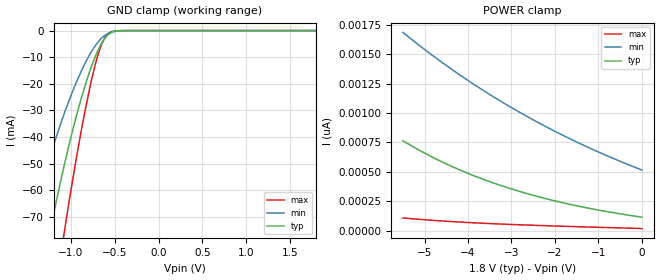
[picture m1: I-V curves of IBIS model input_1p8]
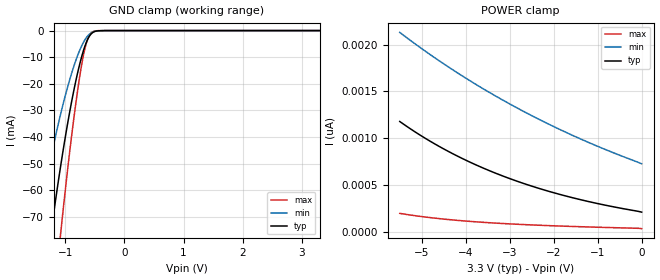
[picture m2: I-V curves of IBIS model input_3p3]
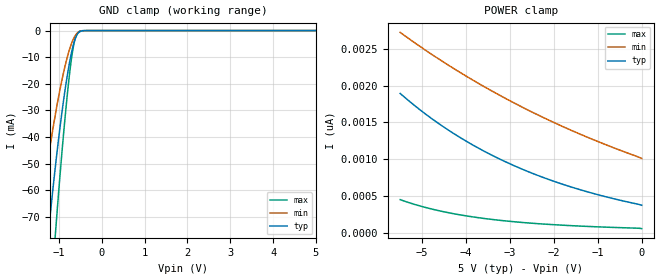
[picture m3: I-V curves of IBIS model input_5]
|Texas Instruments Incorporated
| 2-Bit Bidirectional Voltage-Level Translator with Auto Direction Sensing
| and +/-15-kV ESD Protect
| Marketing part#   Digital Voltage Range   Package-type   #pins
| TXB0102DCTR   1.2V-5.5V   SOT-23   8
| TXB0102DCTT   1.2V-5.5V   SOT-23   8
| TXB0102DCUR   1.2V-5.5V   SOT-70   8
| TXB0102DCUT   1.2V-5.5V   SOT-70   8
| TXB0102YZPR   1.2V-5.5V   WCSP   8
[IBIS Ver]   4.1
[File name]   txb0102.ibs
[File Rev]   2.0
[Date]   5/20/2014
[Source]
| Texas Instruments Incorporated.
| Analog-eLab Design Center, HPA
| 12500 TI Blvd
| Dallas, TX -75243
[Notes]   Revision History:
| Rev 1.0: 2/06/2006
| - Original model based on LVC2T55
| Rev 2.0: 5/20/2014
| - Initial version of the model
| - Model generated from simulations in TISPICE
| - Model matched to SPICE simulation
| - C_comp although listed in numerical order of value are
|   obtained from varying PVT conditions. For PVT conditions for
|   each specific value refer the buffer description under
|   respective [Model]. IBIS model user is responsible for using
|   appropriate C_comp to simulate for Signal Integrity.
| - input_*.ibs models are taken from ibis file available in web.
|* EXCEPTION:   *
|* - For models a_* and b_*, There will be leakage currents in the   *
|*   POWER clamp I-V Table because of two resistors (Ra1 & Rb1)   *
|*   connected to Pad.   *
[Disclaimer]
| This model is designed as an aid for customers of Texas Instruments.
| TI and its licensors and suppliers make no warranties, either expressed
| or implied, with respect to this  model, including the warranties of
| merchantability or fitness for a particular purpose. The model is
| provided solely on an "as is" basis. The entire risk as to its quality
| and performance is with the customer.
[Copyright]
(C) Copyright 2014 Texas Instruments Incorporated.All rights reserved.
|   TXB0102DCT
[Component]   TXB0102DCT
[Manufacturer]   TI
[Package]   |8 SOT-23   -  DCT package
|   typ   min   max
R_pkg   0.02960   0.02800   0.03100
L_pkg   1.85720nH   1.73600nH   1.92400nH
C_pkg   0.22720pF   0.22100pF   0.24200pF
[Pin]  signal_name   model_name   R_pin   L_pin   C_pin
1   B2   B   0.03100   1.89400nH  0.22300pF
2   GND   GND   0.02800   1.69700nH  0.23700pF
3   VCCA   POWER   0.03000   1.72200nH  0.23900pF
4   A2   A   0.03000   1.86100nH  0.22100pF
5   A1   A   0.02800   1.92400nH  0.22800pF
6   OE   OE   0.02900   1.73600nH  0.24200pF
7   VCCB   POWER   0.02800   1.66600nH  0.23600pF
8   B1   B   0.03000   1.87100nH  0.22200pF
|   TXB0102DCU
[Component]   TXB0102DCU
[Manufacturer]   TI
[Package]   |8 SOT-70   -  DCU package
|   typ   min   max
R_pkg   0.02780   0.02300   0.03800
L_pkg   1.58080nH   1.10000nH   2.04600nH
C_pkg   0.28400pF   0.22400pF   0.37200pF
[Pin]  signal_name   model_name   R_pin   L_pin   C_pin
1   B2   B   0.02400   1.52000nH  0.27100pF
2   GND   GND   0.02300   1.11200nH  0.21800pF
3   VCCA   POWER   0.02300   1.07000nH  0.21700pF
4   A2   A   0.02700   2.04600nH  0.37200pF
5   A1   A   0.02700   1.54200nH  0.27300pF
6   OE   OE   0.02300   1.10000nH  0.22400pF
7   VCCB   POWER   0.02300   1.06600nH  0.21500pF
8   B1   B   0.03800   1.69600nH  0.28000pF
|   TXB0102YZP
[Component]   TXB0102YZP
[Manufacturer]   TI
[Package]   |8 WCSP   -  YZP package
|   typ   min   max
R_pkg   0.00100   0.00100   0.00100
L_pkg   0.02480nH   0.02400nH   0.02500nH
C_pkg   0.06460pF   0.06400pF   0.06700pF
[Pin]  signal_name   model_name   R_pin   L_pin   C_pin
A1   B2   B   0.00100   0.02500nH  0.06400pF
B1   GND   GND   0.00100   0.02400nH  0.06700pF
C1   VCCA   POWER   0.00100   0.02400nH  0.06700pF
D1   A2   A   0.00100   0.02500nH  0.06400pF
D2   A1   A   0.00100   0.02500nH  0.06400pF
C2   OE   OE   0.00100   0.02400nH  0.06700pF
B2   VCCB   POWER   0.00100   0.02400nH  0.06700pF
A2   B1   B   0.00100   0.02500nH  0.06400pF
|   Model Selectors
[Model Selector] OE
input_1p8   1.8V  digital Input
input_3p3   3.3V  digital Input
input_5   5.0V  digital Input
[Model Selector] A
a_1p8   1.8V  digital I/O
a_3p3   3.3V  digital I/O
[Model Selector] B
b_1p8   1.8V  digital I/O
b_3p3   3.3V  digital I/O
b_5   5.0V  digital I/O
| Models and submodels in the file (8): input_1p8 (Input), input_3p3 (Input), input_5 (Input), a_1p8 (I/O), a_3p3 (I/O), b_1p8 (I/O), b_3p3 (I/O), b_5 (I/O)
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|   input_1p8 Model
[Model]   input_1p8
Model_type   Input
Vinl = 0.63
Vinh = 1.17
|   typ   min   max
|   (nom PVT)   (fast PVT)   (slow PVT)
C_comp   3.03e-12   2.64e-12   3.31e-12
[Model spec]
|subparameter
Vinl   0.63   0.567   0.693
Vinh   1.17   1.053   1.287
| Where nom  PVT is Nominal Process, 1.8V, 40C
|   Fast PVT is Strong Process,  1.95V, -40C
|   Slow PVT is Weak Process,   1.65V, 100C
[Voltage range]   1.8   1.65   1.95
|Junction Temperature
[Temperature Range]   40   100   -40
[GND Clamp Reference]   0   0   0
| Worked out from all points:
|   GND clamp passes 1 mA (typ) near -0.55 V on its own axis
[GND Clamp]
|   Voltage   I(typ)   I(min)   I(max)
-5.5V     -1.044A    -792.2mA   -1.306A
-1.5V     -120.7mA   -77.56mA   -175.7mA
-1.45V    -111.6mA   -71.36mA   -163.1mA
-1.24V    -75.49mA   -47.29mA   -112.2mA
-1.08V    -50.99mA   -31.4mA    -76.39mA
-1.06V    -48.14mA   -29.58mA   -72.15mA
-920mV    -29.8mA    -17.97mA   -44.33mA
-765mV    -13.32mA   -7.821mA   -18.4mA
-660mV    -5.291mA   -3.146mA   -5.95mA
-575mV    -1.539mA   -1.032mA   -1.212mA
-375mV    -12.62uA   -15.88uA   -2.272uA
1.8V      112.9pA    537.9pA    13.45pA
[POWER Clamp]
|   Voltage   I(typ)   I(min)   I(max)
-5.5V     764.9pA    1.688nA    107.7pA
-4.945V   649pA      1.527nA    90.44pA
-4.36V    543.9pA    1.369nA    76.04pA
-3.745V   449.8pA    1.216nA    63.86pA
-3.09V    365pA      1.067nA    53.22pA
-2.365V   286.8pA    915.8pA    43.31pA
-1.615V   220.2pA    774.7pA    34.41pA
-860mV    165.1pA    646.7pA    26.34pA
-95.1fV   112.9pA    514.9pA    16.24pA
|   input_3p3 Model
[Model]   input_3p3
Model_type   Input
Vinl = 1.155
Vinh = 2.145
|   typ   min   max
|   (nom PVT)   (fast PVT)   (slow PVT)
C_comp   2.89e-12   2.49e-12   3.27e-12
[Model spec]
|subparameter
Vinl   1.155   1.05   1.26
Vinh   2.145   1.95   2.34
| Where nom  PVT is Nominal Process, 3.3V, 40C
|   Fast PVT is Strong Process,  3.6V, -40C
|   Slow PVT is Weak Process,   3V, 100C
[Voltage range]   3.3   3   3.6
|Junction Temperature
[Temperature Range]   40   100   -40
[GND Clamp Reference]   0   0   0
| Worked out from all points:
|   GND clamp passes 1 mA (typ) near -0.55 V on its own axis
[GND Clamp]
|   Voltage   I(typ)   I(min)   I(max)
-5.5V     -1.044A    -792.2mA   -1.306A
-1.49V    -118.9mA   -76.3mA    -173.2mA
-1.245V   -76.3mA    -47.83mA   -113.4mA
-1.085V   -51.71mA   -31.86mA   -77.46mA
-1.065V   -48.85mA   -30.03mA   -73.2mA
-915mV    -29.2mA    -17.6mA    -43.4mA
-755mV    -12.42mA   -7.287mA   -16.97mA
-655mV    -4.994mA   -2.979mA   -5.529mA
-610mV    -2.74mA    -1.719mA   -2.559mA
-545mV    -866.8uA   -625uA     -578.6uA
-325mV    -2.884uA   -4.529uA   -313.3nA
3.3V      208.2pA    781pA      25.79pA
[POWER Clamp]
|   Voltage   I(typ)   I(min)   I(max)
-5.5V     1.179nA    2.132nA    195.3pA
-4.945V   1.006nA    1.94nA     157.6pA
-4.36V    849.7pA    1.752nA    127.8pA
-3.745V   709.5pA    1.569nA    104.1pA
-3.09V    583.3pA    1.39nA     85.02pA
-2.405V   472.8pA    1.219nA    69.68pA
-1.68V    375.8pA    1.054nA    56.89pA
-910mV    291.2pA    895.2pA    45.82pA
-95.1fV   208.2pA    725.8pA    31.68pA
|   input_5 Model
[Model]   input_5
Model_type   Input
Vinl = 1.75
Vinh = 3.25
|   typ   min   max
|   (nom PVT)   (fast PVT)   (slow PVT)
C_comp   2.79e-12   2.38e-12   3.25e-12
[Model spec]
|subparameter
Vinl   1.75   1.575   1.925
Vinh   3.25   2.925   3.575
| Where nom  PVT is Nominal Process, 5V, 40C
|   Fast PVT is Strong Process,  5.5V, -40C
|   Slow PVT is Weak Process,   4.5V, 100C
[Voltage range]   5   4.5   5.5
|Junction Temperature
[Temperature Range]   40   100   -40
[GND Clamp Reference]   0   0   0
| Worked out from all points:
|   GND clamp passes 1 mA (typ) near -0.55 V on its own axis
[GND Clamp]
|   Voltage   I(typ)   I(min)   I(max)
-5.5V     -1.044A    -792.2mA   -1.306A
-1.49V    -118.9mA   -76.3mA    -173.2mA
-1.235V   -74.68mA   -46.76mA   -111.1mA
-1.095V   -53.15mA   -32.79mA   -79.61mA
-1.07V    -49.56mA   -30.49mA   -74.26mA
-890mV    -26.26mA   -15.76mA   -38.86mA
-815mV    -18.12mA   -10.73mA   -26.1mA
-735mV    -10.71mA   -6.271mA   -14.23mA
-675mV    -6.235mA   -3.679mA   -7.319mA
-625mV    -3.404mA   -2.091mA   -3.385mA
-515mV    -456.6uA   -357.2uA   -255.2uA
5V        373.8pA    1.124nA    43.71pA
[POWER Clamp]
|   Voltage   I(typ)   I(min)   I(max)
-5.5V     1.895nA    2.726nA    450.2pA
-4.945V   1.625nA    2.492nA    347.6pA
-4.36V    1.38nA     2.264nA    268pA
-3.745V   1.16nA     2.042nA    207pA
-3.09V    962.2pA    1.824nA    160.3pA
-2.405V   788.8pA    1.615nA    125.4pA
-1.68V    636.5pA    1.414nA    98.78pA
-935mV    507.7pA    1.226nA    78.85pA
-95.1fV   373.8pA    1.011nA    55.56pA
